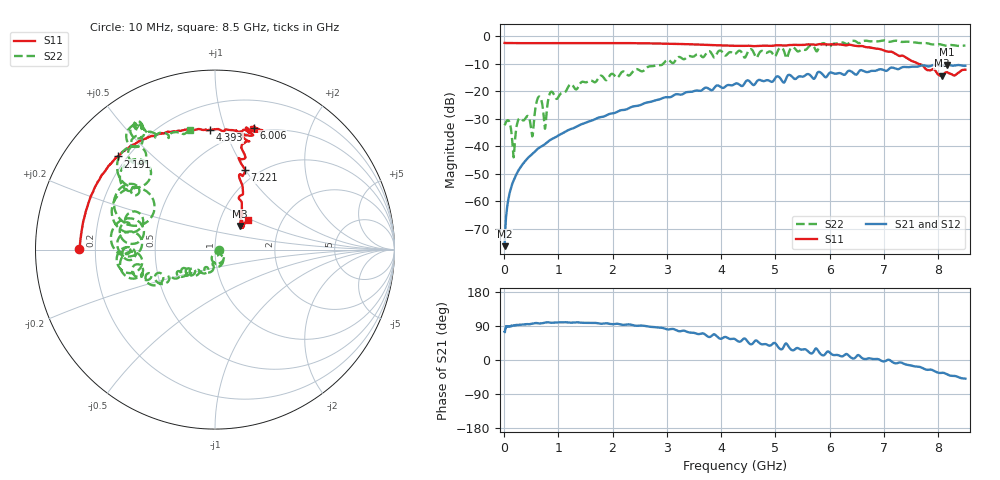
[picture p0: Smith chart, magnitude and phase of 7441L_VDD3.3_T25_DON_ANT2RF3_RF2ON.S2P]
!Agilent Technologies,E5071C,MY46417908,A.11.23
!Date: Mon May 03 19:54:04 2021
!Data & Calibration Information:
!Freq	S11:SOLT2(ON)	S21:SOLT2(ON)	S12:SOLT2(ON)	S22:SOLT2(ON)
!PortZ  Port1:50+j0  Port2:50+j0
!Above PortZ is port z conversion or system Z0 setting when saving the data.
!When reading, reference impedance value at option line is always used.
# Hz S dB R 50
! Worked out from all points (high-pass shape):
!   1601 points, 10 MHz to 8.5 GHz, reference 50 ohm
!   highest |S21| = -10.28 dB at 8.16 GHz (marker M1); lowest = -76.4 dB at 10 MHz (marker M2)
!   |S21| within 3 dB of the highest: 6.31 GHz to 6.43 GHz (120.2 MHz wide, 1.89 % of centre); 6.524 GHz to end of sweep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
!   lowest |S11| = -14.4 dB at 8.065 GHz (marker M3), VSWR 1.47, Z = 63.6 + j17.3 ohm
!   |S11| at or under -10 dB: 7.632 GHz to end of sweep
!   |S22| runs from -44.1 to -1.5 dB; largest |S21 - S12| = 0.0022
!   S11 on the Smith chart (normalised r, x): 10 MHz: 0.14, +0.00; 2.191 GHz: 0.16, +0.39; 4.393 GHz: 0.37, +0.89; 6.006 GHz: 0.46, +1.26; 7.221 GHz: 0.87, +1.00; 8.5 GHz: 1.35, +0.47
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1e7  -2.42 179.7  -76.39 74.2  -76.28 87.1  -32.42 0.3
7.898125e7  -2.47 178.0  -59.31 88.6  -59.40 88.9  -30.57 -33.2
1.798e8  -2.49 175.7  -52.23 90.7  -52.31 90.9  -43.88 -17.7
3.124562e8  -2.51 172.7  -47.43 93.3  -47.39 93.1  -30.00 -43.6
5.140938e8  -2.49 168.2  -42.97 95.9  -42.95 95.9  -36.02 -64.1
6.361375e8  -2.50 165.4  -40.70 96.8  -40.69 96.6  -22.07 -63.7
7.52875e8  -2.49 162.9  -39.27 98.7  -39.30 98.7  -33.65 -81.4
8.643062e8  -2.49 160.4  -37.59 98.4  -37.56 98.5  -20.23 -77.0
1.426769e9  -2.46 149.5  -32.03 98.4  -32.02 98.3  -16.68 -114.7
2.190869e9  -2.49 136.3  -26.84 92.6  -26.84 92.6  -12.83 -143.0
2.843538e9  -2.64 125.6  -23.07 85.5  -23.09 85.5  -10.47 -149.8
4.255e9  -3.49 94.8  -17.30 55.1  -17.30 55.1  -6.50 -178.3
4.392962e9  -3.51 92.2  -18.08 53.5  -18.09 53.4  -6.44 167.8
5.141144e9  -3.33 73.5  -16.74 31.9  -16.72 31.8  -4.67 144.0
5.241962e9  -3.20 74.8  -14.06 35.5  -14.04 35.6  -6.18 164.0
5.671769e9  -3.00 69.2  -14.86 17.5  -14.82 17.3  -3.23 135.6
6.006062e9  -2.96 72.4  -13.23 18.8  -13.22 19.1  -3.73 132.7
7.088538e9  -5.60 74.6  -11.95 0.7  -11.98 0.7  -2.00 121.1
7.221194e9  -6.48 69.3  -11.84 -8.9  -11.85 -9.0  -1.61 121.5
8.064888e9  -14.36 43.2  -10.78 -33.8  -10.79 -33.8  -3.07 112.8
8.1604e9  -13.08 47.1  -10.28 -37.9  -10.33 -38.0  -3.40 112.6
8.5e9  -12.17 41.9  -10.74 -49.2  -10.79 -49.2  -3.37 101.7
